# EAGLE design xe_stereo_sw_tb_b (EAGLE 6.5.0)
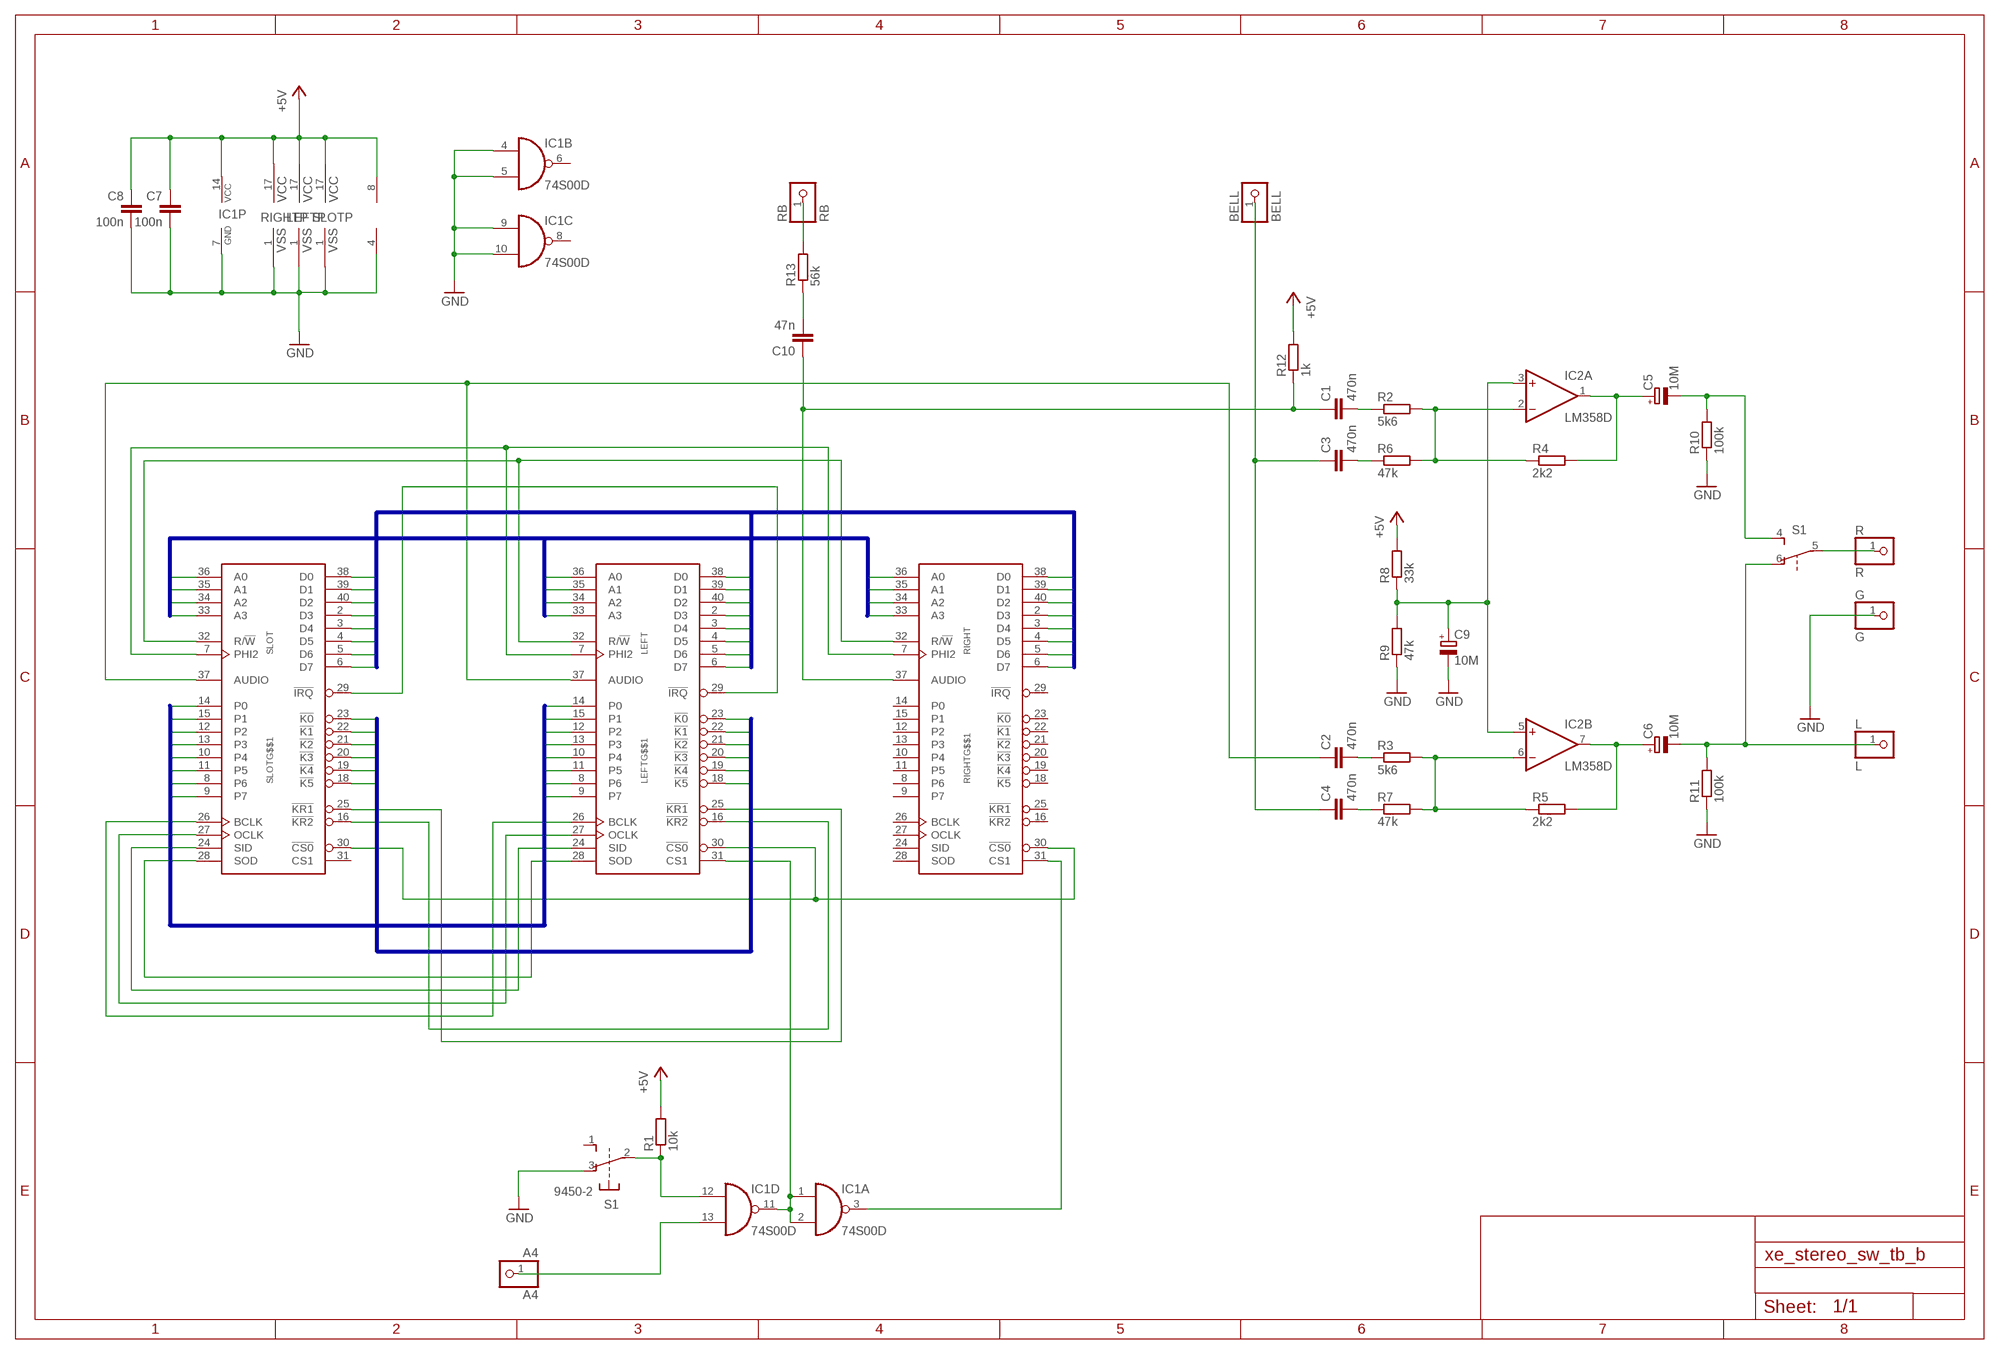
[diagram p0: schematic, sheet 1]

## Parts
A4  A4  PINHD-1X1  [1X01]
BELL  BELL  PINHD-1X1  [1X01]
C1  470n  C-EUC0805  [C0805]
C2  470n  C-EUC0805  [C0805]
C3  470n  C-EUC0805  [C0805]
C4  470n  C-EUC0805  [C0805]
C5  10M  CPOL-EUE2.5-6  [E2,5-6]
C6  10M  CPOL-EUE2.5-6  [E2,5-6]
C7  100n  C-EUC0805  [C0805]
C8  100n  C-EUC0805  [C0805]
C9  10M  CPOL-EUE2.5-6  [E2,5-6]
C10  47n  C-EUC0805  [C0805]
G  G  PINHD-1X1  [1X01]
IC1  74S00D  [SO14]
IC2  LM358D  [SO08]
L  L  PINHD-1X1  [1X01]
LEFT  LEFT  POKEY  [DIL40]
R  R  PINHD-1X1  [1X01]
R1  10k  R-EU_R0805  [R0805]
R2  5k6  R-EU_R0805  [R0805]
R3  5k6  R-EU_R0805  [R0805]
R4  2k2  R-EU_R0805  [R0805]
R5  2k2  R-EU_R0805  [R0805]
R6  47k  R-EU_R0805  [R0805]
R7  47k  R-EU_R0805  [R0805]
R8  33k  R-EU_R0805  [R0805]
R9  47k  R-EU_R0805  [R0805]
R10  100k  R-EU_R0805  [R0805]
R11  100k  R-EU_R0805  [R0805]
R12  1k  R-EU_R0805  [R0805]
R13  56k  R-EU_R0805  [R0805]
RB  RB  PINHD-1X1  [1X01]
RIGHT  RIGHT  POKEY  [DIL40]
S1  9450-2  [9450-2]
SLOT  SLOT  POKEY  [DIL40]

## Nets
+5V: C7.1 C8.1 IC1.14(P:VCC) IC2.8(P:V+) LEFT.17(P:VCC) R1.2 R8.2 R12.2 RIGHT.17(P:VCC) SLOT.17(P:VCC)
A0: LEFT.36(G$$1:A0) RIGHT.36(G$$1:A0) SLOT.36(G$$1:A0)
A1: LEFT.35(G$$1:A1) RIGHT.35(G$$1:A1) SLOT.35(G$$1:A1)
A2: LEFT.34(G$$1:A2) RIGHT.34(G$$1:A2) SLOT.34(G$$1:A2)
A3: LEFT.33(G$$1:A3) RIGHT.33(G$$1:A3) SLOT.33(G$$1:A3)
BELL: BELL.1 C3.1 C4.1
D0: LEFT.38(G$$1:D0) RIGHT.38(G$$1:D0) SLOT.38(G$$1:D0)
D1: LEFT.39(G$$1:D1) RIGHT.39(G$$1:D1) SLOT.39(G$$1:D1)
D2: LEFT.40(G$$1:D2) RIGHT.40(G$$1:D2) SLOT.40(G$$1:D2)
D3: LEFT.2(G$$1:D3) RIGHT.2(G$$1:D3) SLOT.2(G$$1:D3)
D4: LEFT.3(G$$1:D4) RIGHT.3(G$$1:D4) SLOT.3(G$$1:D4)
D5: LEFT.4(G$$1:D5) RIGHT.4(G$$1:D5) SLOT.4(G$$1:D5)
D6: LEFT.5(G$$1:D6) RIGHT.5(G$$1:D6) SLOT.5(G$$1:D6)
D7: LEFT.6(G$$1:D7) RIGHT.6(G$$1:D7) SLOT.6(G$$1:D7)
GND: C7.2 C8.2 C9.- G.1 IC1.4(B:I0) IC1.5(B:I1) IC1.7(P:GND) IC1.9(C:I0) IC1.10(C:I1) IC2.4(P:V-) LEFT.1(P:VSS) R9.1 R10.1 R11.1 RIGHT.1(P:VSS) S1.3(1:O) SLOT.1(P:VSS)
K0: LEFT.23(G$$1:!K0) SLOT.23(G$$1:!K0)
K1: LEFT.22(G$$1:!K1) SLOT.22(G$$1:!K1)
K2: LEFT.21(G$$1:!K2) SLOT.21(G$$1:!K2)
K3: LEFT.20(G$$1:!K3) SLOT.20(G$$1:!K3)
K4: LEFT.19(G$$1:!K4) SLOT.19(G$$1:!K4)
K5: LEFT.18(G$$1:!K5) SLOT.18(G$$1:!K5)
LEFT_OUT: C6.- L.1 R11.2 S1.6(2:O)
N$1: LEFT.30(G$$1:!CS0) RIGHT.30(G$$1:!CS0) SLOT.30(G$$1:!CS0)
N$2: LEFT.29(G$$1:!IRQ) SLOT.29(G$$1:!IRQ)
N$3: A4.1 IC1.13(D:I1)
N$4: LEFT.32(G$$1:R/!W) RIGHT.32(G$$1:R/!W) SLOT.32(G$$1:R/!W)
N$5: IC1.3(A:O) RIGHT.31(G$$1:CS1)
N$6: LEFT.7(G$$1:PHI2) RIGHT.7(G$$1:PHI2) SLOT.7(G$$1:PHI2)
N$7: IC1.1(A:I0) IC1.2(A:I1) IC1.11(D:O) LEFT.31(G$$1:CS1)
N$8: LEFT.28(G$$1:SOD) SLOT.28(G$$1:SOD)
N$9: LEFT.24(G$$1:SID) SLOT.24(G$$1:SID)
N$10: LEFT.27(G$$1:OCLK) SLOT.27(G$$1:OCLK)
N$11: LEFT.26(G$$1:BCLK) SLOT.26(G$$1:BCLK)
N$12: LEFT.16(G$$1:!KR2) SLOT.16(G$$1:!KR2)
N$13: LEFT.25(G$$1:!KR1) SLOT.25(G$$1:!KR1)
N$14: IC1.12(D:I0) R1.1 S1.2(1:P)
N$15: IC2.2(A:-IN) R2.2 R4.1 R6.2
N$16: C1.2 R2.1
N$17: IC2.6(B:-IN) R3.2 R5.1 R7.2
N$18: C2.2 R3.1
N$19: C1.1 C10.1 R12.1 RIGHT.37(G$$1:AUDIO)
N$20: C2.1 LEFT.37(G$$1:AUDIO) SLOT.37(G$$1:AUDIO)
N$21: C5.+ IC2.1(A:OUT) R4.2
N$22: C6.+ IC2.7(B:OUT) R5.2
N$23: R.1 S1.5(2:P)
N$24: C4.2 R7.1
N$25: C3.2 R6.1
N$26: C9.+ IC2.3(A:+IN) IC2.5(B:+IN) R8.1 R9.2
N$27: C10.2 R13.1
N$28: R13.2 RB.1
P0: LEFT.14(G$$1:P0) SLOT.14(G$$1:P0)
P1: LEFT.15(G$$1:P1) SLOT.15(G$$1:P1)
P2: LEFT.12(G$$1:P2) SLOT.12(G$$1:P2)
P3: LEFT.13(G$$1:P3) SLOT.13(G$$1:P3)
P4: LEFT.10(G$$1:P4) SLOT.10(G$$1:P4)
P5: LEFT.11(G$$1:P5) SLOT.11(G$$1:P5)
P6: LEFT.8(G$$1:P6) SLOT.8(G$$1:P6)
P7: LEFT.9(G$$1:P7) SLOT.9(G$$1:P7)
RIGH_OUT: C5.- R10.2 S1.4(2:S)
Unconnected: IC1.6(B:O) IC1.8(C:O) RIGHT.8(G$$1:P6) RIGHT.9(G$$1:P7) RIGHT.10(G$$1:P4) RIGHT.11(G$$1:P5) RIGHT.12(G$$1:P2) RIGHT.13(G$$1:P3) RIGHT.14(G$$1:P0) RIGHT.15(G$$1:P1) RIGHT.16(G$$1:!KR2) RIGHT.18(G$$1:!K5) RIGHT.19(G$$1:!K4) RIGHT.20(G$$1:!K3) RIGHT.21(G$$1:!K2) RIGHT.22(G$$1:!K1) RIGHT.23(G$$1:!K0) RIGHT.24(G$$1:SID) RIGHT.25(G$$1:!KR1) RIGHT.26(G$$1:BCLK) RIGHT.27(G$$1:OCLK) RIGHT.28(G$$1:SOD) RIGHT.29(G$$1:!IRQ) S1.1(1:S) SLOT.31(G$$1:CS1)

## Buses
A[0..3]
D[0..7]
P[0..7]
K[0..5]

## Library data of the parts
A4 BELL G L R RB = pinhead:PINHD-1X1: PIN HEADER
C1-C4 C7 C8 C10 = rcl:C-EU: CAPACITOR, European symbol
C5 C6 C9 = rcl:CPOL-EU: POLARIZED CAPACITOR, European symbol
IC1 = 74xx-eu:74*00: Quad 2-input NAND gate
IC2 = linear:LM358: OP AMP also LM158; LM258; LM2904 Source: http://cache.national.com/ds/LM/LM158.pdf
LEFT RIGHT SLOT = eagle-6.5.0-atari:POKEY: POKEY
R1-R13 = rcl:R-EU_: RESISTOR, European symbol
S1 = switch-misc:9450-2: MARQUARDT SWITCH

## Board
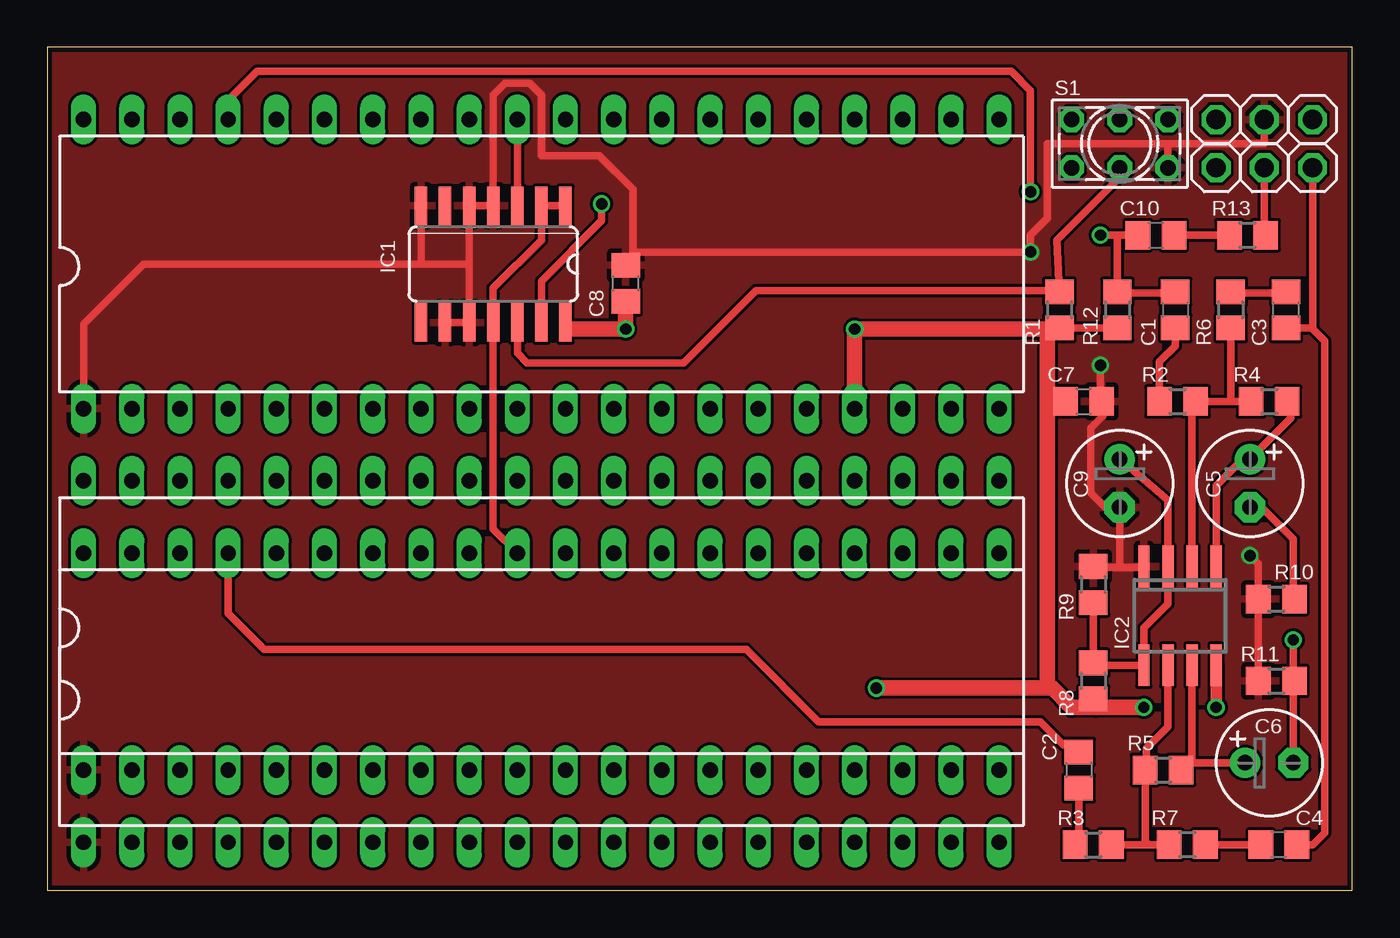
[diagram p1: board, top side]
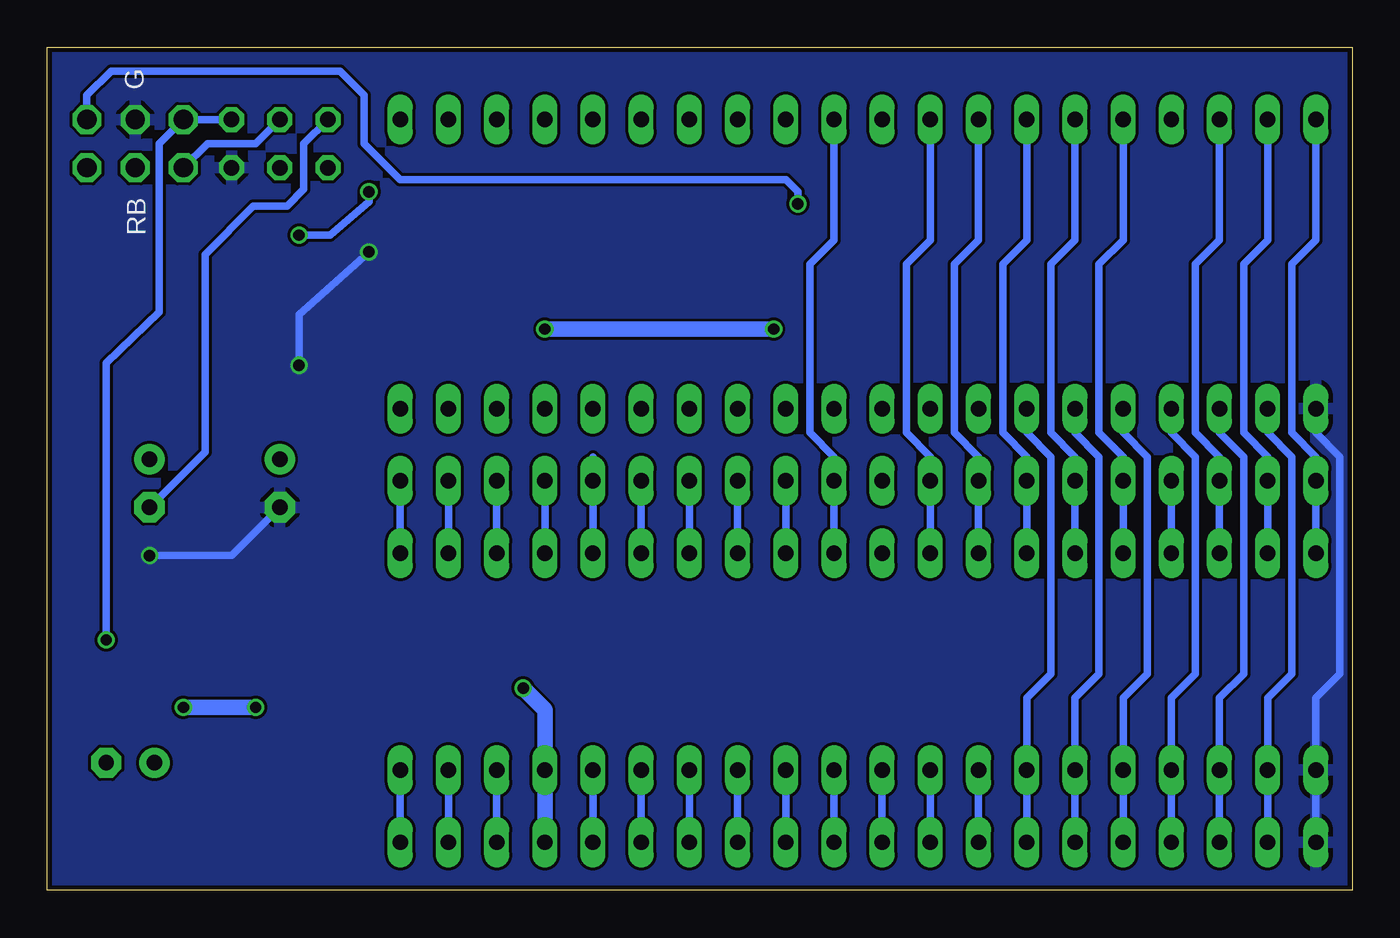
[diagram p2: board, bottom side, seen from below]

Size 68.76 x 44.44 mm. Coordinates in mm from the lower left corner, seen from the top.
Outline: 0,0 68.76,0 68.76,44.44 0,44.44 0,0
Copper layers (1*16): Top 0.035mm / dielectric 1.5mm / Bottom 0.035mm
Design rules "SeeedStudio_2layer_DRU_no_angle_20140221": minimum track width 6mil, minimum drill 12mil, track to track 6mil, track to pad 6mil, pad to pad 6mil, via to via 6mil, smd to smd 0mil, copper to edge 10mil, drill to drill 10mil, minimum pad ring 10mil, minimum via ring 6mil, stop-mask expansion 2mil, vias tented up to drill 100mil, thermal gap 10mil

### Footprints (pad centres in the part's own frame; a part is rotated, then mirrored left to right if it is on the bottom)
1X01 = drill 1.016 octagon: 1 0,0
C0805 = smd 1.3 x 1.5: 1 -0.95,0; 2 0.95,0
E2,5-6 = drill 0.813 pad 1.6: + -1.27,0 | drill 0.813 pad 1.6 octagon: - 1.27,0
SO14 = smd 0.66 x 2.032: 1 -3.81,-3.073; 2 -2.54,-3.073; 3 -1.27,-3.073; 4 0,-3.073; 5 1.27,-3.073; 6 2.54,-3.073; 7 3.81,-3.073; 8 3.81,3.073; 9 2.54,3.073; 10 1.27,3.073; 11 0,3.073; 12 -1.27,3.073; 13 -2.54,3.073; 14 -3.81,3.073
SO08 = smd 0.6 x 2.2: 1 -1.905,-2.6; 2 -0.635,-2.6; 3 0.635,-2.6; 4 1.905,-2.6; 5 1.905,2.6; 6 0.635,2.6; 7 -0.635,2.6; 8 -1.905,2.6
DIL40 = drill 0.813 long: 1 -24.13,-7.62; 2 -21.59,-7.62; 3 -19.05,-7.62; 4 -16.51,-7.62; 5 -13.97,-7.62; 6 -11.43,-7.62; 7 -8.89,-7.62; 8 -6.35,-7.62; 9 -3.81,-7.62; 10 -1.27,-7.62; 11 1.27,-7.62; 12 3.81,-7.62; 13 6.35,-7.62; 14 8.89,-7.62; 15 11.43,-7.62; 16 13.97,-7.62; 17 16.51,-7.62; 18 19.05,-7.62; 19 21.59,-7.62; 20 24.13,-7.62; 21 24.13,7.62; 22 21.59,7.62; 23 19.05,7.62; 24 16.51,7.62; 25 13.97,7.62; 26 11.43,7.62; 27 8.89,7.62; 28 6.35,7.62; 29 3.81,7.62; 30 1.27,7.62; 31 -1.27,7.62; 32 -3.81,7.62; 33 -6.35,7.62; 34 -8.89,7.62; 35 -11.43,7.62; 36 -13.97,7.62; 37 -16.51,7.62; 38 -19.05,7.62; 39 -21.59,7.62; 40 -24.13,7.62
R0805 = smd 1.3 x 1.5: 1 -0.95,0; 2 0.95,0
9450-2 = drill 0.813 octagon: 1 -2.54,-1.27; 2 0,-1.27; 3 2.54,-1.27; 4 -2.54,1.27; 5 0,1.27; 6 2.54,1.27

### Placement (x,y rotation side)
A4  66.68,40.64 180 top
BELL  66.68,38.1 180 top
C1  59.44,30.61 270 top
C2  54.36,6.35 270 top
C3  65.28,30.61 90 top
C4  64.9,2.41 180 top
C5  63.37,21.46 270 top
C6  64.39,6.73 0 top
C7  54.61,25.78 0 top
C8  30.48,32 90 top
C9  56.51,21.46 270 top
C10  58.42,34.54 0 top
G  64.13,40.64 0 top
IC1  23.49,33.02 180 top
IC2  59.69,14.48 180 top
L  61.59,40.64 180 top
LEFT  26.03,10.16 0 top
R  61.59,38.1 180 top
R1  53.34,30.61 270 top
R2  59.56,25.78 0 top
R3  55.12,2.41 0 top
R4  64.39,25.78 0 top
R5  58.8,6.35 0 top
R6  62.36,30.61 270 top
R7  60.07,2.41 180 top
R8  55.12,11.05 270 top
R9  55.12,16.13 270 top
R10  64.77,15.37 0 top
R11  64.77,11.05 0 top
R12  56.39,30.61 270 top
R13  63.25,34.54 0 top
RB  64.13,38.1 0 top
RIGHT  26.03,33.02 0 top
S1  56.51,39.37 0 top
SLOT  26.03,13.97 0 top

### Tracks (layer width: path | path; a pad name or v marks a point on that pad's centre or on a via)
+5V  (via drill 0.6)
  Top 0.406: 52.77,29.46 R1.2 R12.2 | R8.2 55.12,9.78 55.24,9.65
  Top 0.61: 27.41,29.59 IC1.14 | R1.2 53.21,29.46 52.77,29.21 | v61.59,9.65 IC2.8
  Top 0.813: C8.1 v30.48,29.59 27.41,29.59 | v43.69,10.67 52.71,10.67 | RIGHT.17 v42.54,29.59 52.71,29.59 | 52.77,29.46 52.77,29.21 52.71,29.59 | 52.71,29.59 52.71,25.78 | 52.71,25.78 52.71,10.67 | v57.79,9.65 55.24,9.65 53.98,9.65 52.96,10.67 52.71,10.67 | C7.1 52.71,25.78
  Bottom 0.813: LEFT.17 SLOT.17 42.54,9.53 v43.69,10.67 | v42.54,29.59 v30.48,29.59 | v57.79,9.65 v61.59,9.65
A0
  Bottom 0.406: LEFT.36 SLOT.36 12.06,22.86 13.34,24.13 13.34,33.02 12.06,34.29 RIGHT.36
A1
  Bottom 0.406: LEFT.35 SLOT.35 14.6,22.86 15.88,24.13 15.88,33.02 14.6,34.29 RIGHT.35
A2
  Bottom 0.406: LEFT.34 SLOT.34 17.14,22.86 18.41,24.13 18.41,33.02 17.14,34.29 RIGHT.34
A3
  Bottom 0.406: LEFT.33 SLOT.33 19.68,22.86 20.95,24.13 20.95,33.02 19.68,34.29 RIGHT.33
BELL
  Top 0.406: BELL.1 66.68,29.59 | 66.68,29.59 67.31,28.96 67.31,3.05 66.68,2.41 C4.1 | C3.1 66.61,29.66 66.68,29.59
D0
  Bottom 0.406: RIGHT.38 6.98,34.29 8.25,33.02 8.25,24.13 6.98,22.86 SLOT.38 LEFT.38
D1
  Bottom 0.406: RIGHT.39 4.45,34.29 5.71,33.02 5.71,24.13 4.45,22.86 SLOT.39 LEFT.39
D2
  Bottom 0.406: SLOT.40 LEFT.40 1.9,22.86 3.17,24.13 3.17,33.02 1.9,34.29 RIGHT.40
D3
  Bottom 0.406: RIGHT.2 4.45,24.13 3.17,22.86 3.17,11.43 4.45,10.16 SLOT.2 LEFT.2
D4
  Bottom 0.406: RIGHT.3 6.98,24.13 5.71,22.86 5.71,11.43 6.98,10.16 SLOT.3 LEFT.3
D5
  Bottom 0.406: RIGHT.4 9.52,24.13 8.25,22.86 8.25,11.43 9.52,10.16 SLOT.4 LEFT.4
D6
  Bottom 0.406: LEFT.5 SLOT.5 12.06,10.16 10.8,11.43 10.8,22.86 12.06,24.13 RIGHT.5
D7
  Bottom 0.406: LEFT.6 SLOT.6 14.6,10.16 13.34,11.43 13.34,22.86 14.6,24.13 RIGHT.6
GND  (via drill 0.6)
  Top 0.406: RIGHT.1 1.9,29.84 5.08,33.02 19.68,33.02 | 22.23,33.02 IC1.10 IC1.9 | 22.23,33.02 IC1.5 IC1.4 23.49,41.91 24.13,42.54 25.4,42.54 26.03,41.91 26.03,38.73 29.08,38.73 30.86,36.96 30.86,33.65 | 19.68,33.65 IC1.7 19.68,33.02 | 19.68,33.02 22.23,33.02 | R11.1 R10.1 63.82,17.21 v63.37,17.65 | C8.2 30.86,33.65 | 30.86,33.65 v51.82,33.65 51.82,34.54 52.71,35.43 52.71,39.37 59.05,39.37 | S1.3 59.05,39.37 | 59.05,39.37 64.13,39.37 G.1 | v55.5,27.69 55.5,25.59 C7.2 | 55.5,25.46 C7.2 | C7.2 55.63,25.02 54.99,24.38 54.99,20.96 55.75,20.19 C9.- 56.51,17.02 | R9.1 55.12,17.02 56.51,17.02 | 56.51,17.02 57.79,17.02 IC2.4
  Bottom 0.406: RIGHT.1 1.9,24.13 0.63,22.86 0.63,11.43 1.9,10.16 SLOT.1 LEFT.1 | v51.82,33.65 55.5,30.35 v55.5,27.69 | v63.37,17.65 59.05,17.65 C9.-
  pour Bottom: -5.71,50.16 71.25,50.16 71.25,-2.54 -5.71,-2.54
  pour Top: -3.81,48.26 72.9,48.26 72.9,-4.45 -3.81,-4.45
K0
  Bottom 0.406: LEFT.23 SLOT.23
K1
  Bottom 0.406: LEFT.22 SLOT.22
K2
  Bottom 0.406: LEFT.21 SLOT.21
K3
  Bottom 0.406: LEFT.20 SLOT.20
K4
  Bottom 0.406: SLOT.19 LEFT.19
K5
  Bottom 0.406: LEFT.18 SLOT.18
LEFT_OUT  (via drill 0.6)
  Top 0.406: v65.66,13.21 65.66,10.98 | 65.66,10.98 R11.2 | C6.- 65.66,10.98
  Bottom 0.406: v65.66,13.21 65.66,27.81 62.87,30.48 62.87,39.37 L.1 S1.6
N$1
  Bottom 0.406: LEFT.30 SLOT.30 27.3,22.86 28.57,24.13 28.57,33.02 27.3,34.29 RIGHT.30
N$2
  Bottom 0.406: SLOT.29 LEFT.29
N$3  (via drill 0.6)
  Top 0.406: IC1.13 26.03,32.13 29.21,35.31 v29.21,36.2
  Bottom 0.406: v29.21,36.2 29.21,36.83 29.84,37.46 50.16,37.46 52.07,39.37 52.07,41.91 53.34,43.18 65.41,43.18 66.68,41.91 A4.1
N$4
  Bottom 0.406: LEFT.32 SLOT.32 22.23,22.86 23.49,24.13 23.49,33.02 22.23,34.29 RIGHT.32
N$5
  Top 0.406: RIGHT.31 IC1.3
N$6
  Bottom 0.406: LEFT.7 SLOT.7 17.14,10.16 15.88,11.43 15.88,22.86 17.14,24.13 RIGHT.7
N$7
  Top 0.406: LEFT.31 23.49,19.05 IC1.11 23.49,31.75 26.03,34.29 IC1.2 IC1.1
N$8
  Bottom 0.406: LEFT.28 SLOT.28
N$9
  Bottom 0.406: LEFT.24 SLOT.24
N$10
  Bottom 0.406: SLOT.27 LEFT.27
N$11
  Bottom 0.406: LEFT.26 SLOT.26
N$12
  Bottom 0.406: SLOT.16 LEFT.16
N$13
  Bottom 0.406: LEFT.25 SLOT.25 40,22.86
N$14
  Top 0.406: IC1.12 24.77,28.32 25.27,27.81 33.53,27.81 37.34,31.62 52.89,31.62 R1.1 53.21,34.29 56.51,37.59 S1.2
N$15
  Top 0.406: IC2.2 60.32,25.78 R2.2 62.36,25.78 | R4.1 62.36,25.78 | R6.2 62.36,25.78
N$16
  Top 0.406: R2.1 58.61,27.88 59.44,28.7 C1.2
N$17
  Top 0.406: R3.2 58.04,2.41 | 58.04,2.41 R7.2 | 58.04,2.41 57.85,2.6 R5.1 57.91,6.41 57.91,7.49 59.05,8.64 IC2.6
N$18
  Top 0.406: 54.29,2.67 R3.1 54.36,3.05 C2.2
N$19  (via drill 0.6)
  Top 0.406: RIGHT.37 9.52,41.66 11.05,43.18 50.8,43.18 51.82,42.16 v51.82,36.83 | C10.1 56.39,34.54 | v55.5,34.54 56.39,34.54 | 56.39,34.54 R12.1 56.39,31.5 58.99,31.5 C1.1
  Bottom 0.406: v51.82,36.83 51.82,36.32 53.85,34.54 v55.5,34.54
N$20
  Top 0.406: C2.1 54.36,7.68 54.48,7.62 53.53,7.68 52.32,8.89 40.64,8.89 36.83,12.7 11.43,12.7 9.52,14.61 LEFT.37
  Bottom 0.406: SLOT.37 LEFT.37
N$21
  Top 0.406: IC2.1 61.59,21.34 62.99,22.73 C5.+ 65.53,24.89 65.53,25.72 R4.2
N$22
  Top 0.406: R5.2 60.2,6.73 60.32,6.73 | 60.32,6.73 C6.+ | IC2.7 60.32,6.73
N$23
  Bottom 0.406: S1.5 57.79,39.37 60.32,39.37 R.1
N$24
  Top 0.406: C4.2 R7.1
N$25
  Top 0.406: R6.1 62.48,31.5 65.09,31.5 C3.2
N$26
  Top 0.406: R9.2 R8.1 55.62,11.88 IC2.5 57.79,13.84 59.05,15.11 IC2.3 59.05,20.57 C9.+
N$27
  Top 0.406: C10.2 R13.1
N$28
  Top 0.406: RB.1 64.13,34.6 R13.2
P0
  Bottom 0.406: SLOT.14 LEFT.14
P1
  Bottom 0.406: LEFT.15 SLOT.15
P2
  Bottom 0.406: SLOT.12 LEFT.12
P3
  Bottom 0.406: LEFT.13 SLOT.13
P4
  Bottom 0.406: SLOT.10 LEFT.10
P5
  Bottom 0.406: LEFT.11 SLOT.11
P6
  Bottom 0.406: SLOT.8 LEFT.8
P7
  Bottom 0.406: LEFT.9 SLOT.9
RIGH_OUT
  Top 0.406: 65.41,15.43 R10.2 65.66,15.43 65.66,18.54 64.01,20.19 C5.-
  Bottom 0.406: S1.4 55.24,39.37 55.24,36.96 56.13,36.07 57.91,36.07 60.45,33.53 60.45,23.11 C5.- 63.25,20.19

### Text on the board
tDocu: RIGHT | SLOT | ATARI STEREO | LEFT | PCB Krupkaj 2017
